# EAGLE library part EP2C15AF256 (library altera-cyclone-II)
EP2C15AF256 Auto generated by make-symbol-device-package-bsdl.ulp Rev. 18 Tip: Use split-device-symbol.ulp to generate a Device with multiple small symbols! Read HELP. Source: EP2C15AF256.BSD
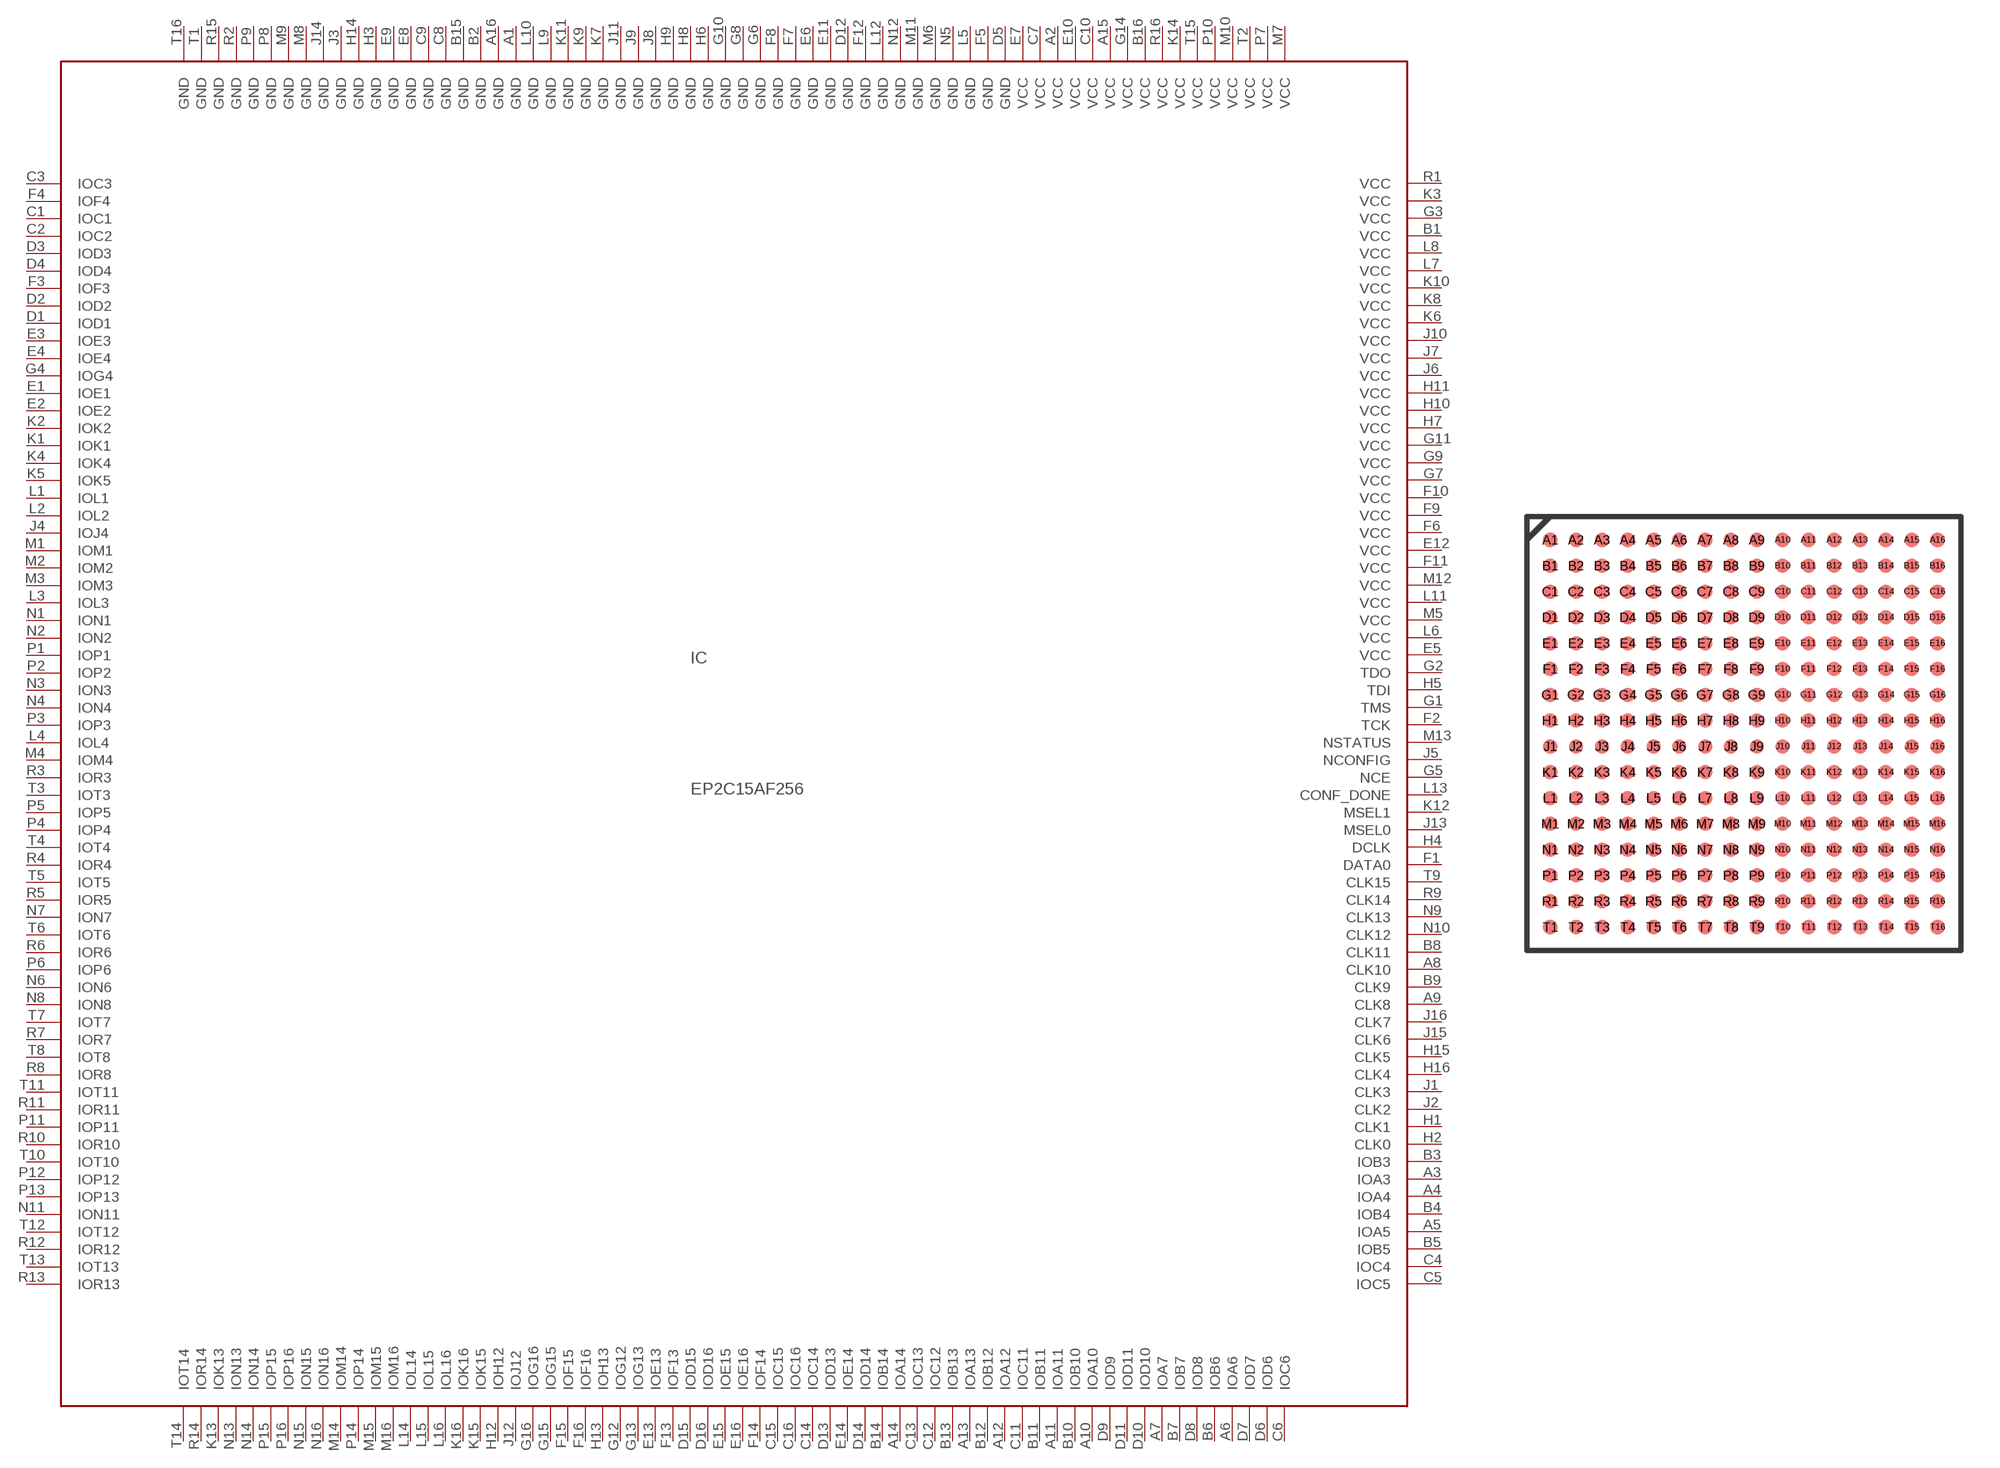
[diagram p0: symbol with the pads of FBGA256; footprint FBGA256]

Designator prefix IC

## EP2C15AF256 (MPN: EP2C15AF256C8N; OC_FARNELL: 1549347; OC_NEWARK: 52R0488)  [FBGA256]
A1  GND  pwr
A2  VCC  pwr
A3  IOA3
A4  IOA4
A5  IOA5
A6  IOA6
A7  IOA7
A8  CLK10
A9  CLK8
A10  IOA10
A11  IOA11
A12  IOA12
A13  IOA13
A14  IOA14
A15  VCC  pwr
A16  GND  pwr
B1  VCC  pwr
B2  GND  pwr
B3  IOB3
B4  IOB4
B5  IOB5
B6  IOB6
B7  IOB7
B8  CLK11
B9  CLK9
B10  IOB10
B11  IOB11
B12  IOB12
B13  IOB13
B14  IOB14
B15  GND  pwr
B16  VCC  pwr
C1  IOC1
C2  IOC2
C3  IOC3  out
C4  IOC4
C5  IOC5
C6  IOC6
C7  VCC  pwr
C8  GND  pwr
C9  GND  pwr
C10  VCC  pwr
C11  IOC11
C12  IOC12
C13  IOC13
C14  IOC14
C15  IOC15
C16  IOC16
D1  IOD1
D2  IOD2
D3  IOD3
D4  IOD4
D5  GND  pwr
D6  IOD6
D7  IOD7
D8  IOD8
D9  IOD9
D10  IOD10
D11  IOD11
D12  GND  pwr
D13  IOD13
D14  IOD14
D15  IOD15
D16  IOD16
E1  IOE1
E2  IOE2
E3  IOE3
E4  IOE4
E5  VCC  pwr
E6  GND  pwr
E7  VCC  pwr
E8  GND  pwr
E9  GND  pwr
E10  VCC  pwr
E11  GND  pwr
E12  VCC  pwr
E13  IOE13
E14  IOE14
E15  IOE15
E16  IOE16
F1  DATA0
F2  TCK  in
F3  IOF3
F4  IOF4  out
F5  GND  pwr
F6  VCC  pwr
F7  GND  pwr
F8  GND  pwr
F9  VCC  pwr
F10  VCC  pwr
F11  VCC  pwr
F12  GND  pwr
F13  IOF13
F14  IOF14
F15  IOF15
F16  IOF16
G1  TMS  in
G2  TDO  out
G3  VCC  pwr
G4  IOG4
G5  NCE  in
G6  GND  pwr
G7  VCC  pwr
G8  GND  pwr
G9  VCC  pwr
G10  GND  pwr
G11  VCC  pwr
G12  IOG12
G13  IOG13
G14  VCC  pwr
G15  IOG15
G16  IOG16
H1  CLK1
H2  CLK0
H3  GND  pwr
H4  DCLK
H5  TDI  in
H6  GND  pwr
H7  VCC  pwr
H8  GND  pwr
H9  GND  pwr
H10  VCC  pwr
H11  VCC  pwr
H12  IOH12
H13  IOH13
H14  GND  pwr
H15  CLK5
H16  CLK4
J1  CLK3
J2  CLK2
J3  GND  pwr
J4  IOJ4
J5  NCONFIG  in
J6  VCC  pwr
J7  VCC  pwr
J8  GND  pwr
J9  GND  pwr
J10  VCC  pwr
J11  GND  pwr
J12  IOJ12
J13  MSEL0  in
J14  GND  pwr
J15  CLK6
J16  CLK7
K1  IOK1
K2  IOK2
K3  VCC  pwr
K4  IOK4
K5  IOK5
K6  VCC  pwr
K7  GND  pwr
K8  VCC  pwr
K9  GND  pwr
K10  VCC  pwr
K11  GND  pwr
K12  MSEL1  in
K13  IOK13
K14  VCC  pwr
K15  IOK15
K16  IOK16
L1  IOL1
L2  IOL2
L3  IOL3
L4  IOL4
L5  GND  pwr
L6  VCC  pwr
L7  VCC  pwr
L8  VCC  pwr
L9  GND  pwr
L10  GND  pwr
L11  VCC  pwr
L12  GND  pwr
L13  CONF_DONE  in
L14  IOL14
L15  IOL15
L16  IOL16
M1  IOM1
M2  IOM2
M3  IOM3
M4  IOM4
M5  VCC  pwr
M6  GND  pwr
M7  VCC  pwr
M8  GND  pwr
M9  GND  pwr
M10  VCC  pwr
M11  GND  pwr
M12  VCC  pwr
M13  NSTATUS  in
M14  IOM14
M15  IOM15
M16  IOM16
N1  ION1
N2  ION2
N3  ION3
N4  ION4
N5  GND  pwr
N6  ION6
N7  ION7
N8  ION8
N9  CLK13
N10  CLK12
N11  ION11
N12  GND  pwr
N13  ION13
N14  ION14
N15  ION15
N16  ION16
P1  IOP1
P2  IOP2
P3  IOP3
P4  IOP4
P5  IOP5
P6  IOP6
P7  VCC  pwr
P8  GND  pwr
P9  GND  pwr
P10  VCC  pwr
P11  IOP11
P12  IOP12
P13  IOP13
P14  IOP14
P15  IOP15
P16  IOP16
R1  VCC  pwr
R2  GND  pwr
R3  IOR3
R4  IOR4
R5  IOR5
R6  IOR6
R7  IOR7
R8  IOR8
R9  CLK14
R10  IOR10
R11  IOR11
R12  IOR12
R13  IOR13
R14  IOR14
R15  GND  pwr
R16  VCC  pwr
T1  GND  pwr
T2  VCC  pwr
T3  IOT3
T4  IOT4
T5  IOT5
T6  IOT6
T7  IOT7
T8  IOT8
T9  CLK15
T10  IOT10
T11  IOT11
T12  IOT12
T13  IOT13
T14  IOT14
T15  VCC  pwr
T16  GND  pwr

## Footprint FBGA256 (pad centres in mm)
EP2C15AF256 Auto generated by make-symbol-device-package-bsdl.ulp Rev. 18 Source: EP2C15AF256.BSD www.altera.com .. cyc2_cii51015.pdf
smd 0.55 x 0.55: A1 -7.5,7.5; A2 -6.5,7.5; A3 -5.5,7.5; A4 -4.5,7.5; A5 -3.5,7.5; A6 -2.5,7.5; A7 -1.5,7.5; A8 -0.5,7.5; A9 0.5,7.5; A10 1.5,7.5; A11 2.5,7.5; A12 3.5,7.5; A13 4.5,7.5; A14 5.5,7.5; A15 6.5,7.5; A16 7.5,7.5; B1 -7.5,6.5; B2 -6.5,6.5; B3 -5.5,6.5; B4 -4.5,6.5; B5 -3.5,6.5; B6 -2.5,6.5; B7 -1.5,6.5; B8 -0.5,6.5; B9 0.5,6.5; B10 1.5,6.5; B11 2.5,6.5; B12 3.5,6.5; B13 4.5,6.5; B14 5.5,6.5; B15 6.5,6.5; B16 7.5,6.5; C1 -7.5,5.5; C2 -6.5,5.5; C3 -5.5,5.5; C4 -4.5,5.5; C5 -3.5,5.5; C6 -2.5,5.5; C7 -1.5,5.5; C8 -0.5,5.5; C9 0.5,5.5; C10 1.5,5.5; C11 2.5,5.5; C12 3.5,5.5; C13 4.5,5.5; C14 5.5,5.5; C15 6.5,5.5; C16 7.5,5.5; D1 -7.5,4.5; D2 -6.5,4.5; D3 -5.5,4.5; D4 -4.5,4.5; D5 -3.5,4.5; D6 -2.5,4.5; D7 -1.5,4.5; D8 -0.5,4.5; D9 0.5,4.5; D10 1.5,4.5; D11 2.5,4.5; D12 3.5,4.5; D13 4.5,4.5; D14 5.5,4.5; D15 6.5,4.5; D16 7.5,4.5; E1 -7.5,3.5; E2 -6.5,3.5; E3 -5.5,3.5; E4 -4.5,3.5; E5 -3.5,3.5; E6 -2.5,3.5; E7 -1.5,3.5; E8 -0.5,3.5; E9 0.5,3.5; E10 1.5,3.5; E11 2.5,3.5; E12 3.5,3.5; E13 4.5,3.5; E14 5.5,3.5; E15 6.5,3.5; E16 7.5,3.5; F1 -7.5,2.5; F2 -6.5,2.5; F3 -5.5,2.5; F4 -4.5,2.5; F5 -3.5,2.5; F6 -2.5,2.5; F7 -1.5,2.5; F8 -0.5,2.5; F9 0.5,2.5; F10 1.5,2.5; F11 2.5,2.5; F12 3.5,2.5; F13 4.5,2.5; F14 5.5,2.5; F15 6.5,2.5; F16 7.5,2.5; G1 -7.5,1.5; G2 -6.5,1.5; G3 -5.5,1.5; G4 -4.5,1.5; G5 -3.5,1.5; G6 -2.5,1.5; G7 -1.5,1.5; G8 -0.5,1.5; G9 0.5,1.5; G10 1.5,1.5; G11 2.5,1.5; G12 3.5,1.5; G13 4.5,1.5; G14 5.5,1.5; G15 6.5,1.5; G16 7.5,1.5; H1 -7.5,0.5; H2 -6.5,0.5; H3 -5.5,0.5; H4 -4.5,0.5; H5 -3.5,0.5; H6 -2.5,0.5; H7 -1.5,0.5; H8 -0.5,0.5; H9 0.5,0.5; H10 1.5,0.5; H11 2.5,0.5; H12 3.5,0.5; H13 4.5,0.5; H14 5.5,0.5; H15 6.5,0.5; H16 7.5,0.5; J1 -7.5,-0.5; J2 -6.5,-0.5; J3 -5.5,-0.5; J4 -4.5,-0.5; J5 -3.5,-0.5; J6 -2.5,-0.5; J7 -1.5,-0.5; J8 -0.5,-0.5; J9 0.5,-0.5; J10 1.5,-0.5; J11 2.5,-0.5; J12 3.5,-0.5; J13 4.5,-0.5; J14 5.5,-0.5; J15 6.5,-0.5; J16 7.5,-0.5; K1 -7.5,-1.5; K2 -6.5,-1.5; K3 -5.5,-1.5; K4 -4.5,-1.5; K5 -3.5,-1.5; K6 -2.5,-1.5; K7 -1.5,-1.5; K8 -0.5,-1.5; K9 0.5,-1.5; K10 1.5,-1.5; K11 2.5,-1.5; K12 3.5,-1.5; K13 4.5,-1.5; K14 5.5,-1.5; K15 6.5,-1.5; K16 7.5,-1.5; L1 -7.5,-2.5; L2 -6.5,-2.5; L3 -5.5,-2.5; L4 -4.5,-2.5; L5 -3.5,-2.5; L6 -2.5,-2.5; L7 -1.5,-2.5; L8 -0.5,-2.5; L9 0.5,-2.5; L10 1.5,-2.5; L11 2.5,-2.5; L12 3.5,-2.5; L13 4.5,-2.5; L14 5.5,-2.5; L15 6.5,-2.5; L16 7.5,-2.5; M1 -7.5,-3.5; M2 -6.5,-3.5; M3 -5.5,-3.5; M4 -4.5,-3.5; M5 -3.5,-3.5; M6 -2.5,-3.5; M7 -1.5,-3.5; M8 -0.5,-3.5; M9 0.5,-3.5; M10 1.5,-3.5; M11 2.5,-3.5; M12 3.5,-3.5; M13 4.5,-3.5; M14 5.5,-3.5; M15 6.5,-3.5; M16 7.5,-3.5; N1 -7.5,-4.5; N2 -6.5,-4.5; N3 -5.5,-4.5; N4 -4.5,-4.5; N5 -3.5,-4.5; N6 -2.5,-4.5; N7 -1.5,-4.5; N8 -0.5,-4.5; N9 0.5,-4.5; N10 1.5,-4.5; N11 2.5,-4.5; N12 3.5,-4.5; N13 4.5,-4.5; N14 5.5,-4.5; N15 6.5,-4.5; N16 7.5,-4.5; P1 -7.5,-5.5; P2 -6.5,-5.5; P3 -5.5,-5.5; P4 -4.5,-5.5; P5 -3.5,-5.5; P6 -2.5,-5.5; P7 -1.5,-5.5; P8 -0.5,-5.5; P9 0.5,-5.5; P10 1.5,-5.5; P11 2.5,-5.5; P12 3.5,-5.5; P13 4.5,-5.5; P14 5.5,-5.5; P15 6.5,-5.5; P16 7.5,-5.5; R1 -7.5,-6.5; R2 -6.5,-6.5; R3 -5.5,-6.5; R4 -4.5,-6.5; R5 -3.5,-6.5; R6 -2.5,-6.5; R7 -1.5,-6.5; R8 -0.5,-6.5; R9 0.5,-6.5; R10 1.5,-6.5; R11 2.5,-6.5; R12 3.5,-6.5; R13 4.5,-6.5; R14 5.5,-6.5; R15 6.5,-6.5; R16 7.5,-6.5; T1 -7.5,-7.5; T2 -6.5,-7.5; T3 -5.5,-7.5; T4 -4.5,-7.5; T5 -3.5,-7.5; T6 -2.5,-7.5; T7 -1.5,-7.5; T8 -0.5,-7.5; T9 0.5,-7.5; T10 1.5,-7.5; T11 2.5,-7.5; T12 3.5,-7.5; T13 4.5,-7.5; T14 5.5,-7.5; T15 6.5,-7.5; T16 7.5,-7.5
